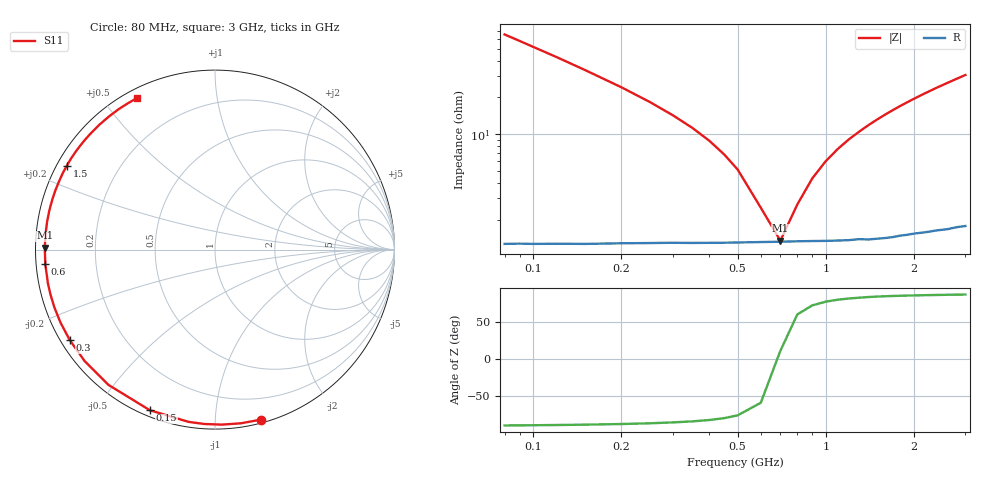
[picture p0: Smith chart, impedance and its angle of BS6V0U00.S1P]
! SIEMENS Small Signal Semiconductors
! BB640
! Si Tuning Diode in SOD323
! VR = 6 V
! S-Parameters:  July  1993
# GHz  S  MA  R  50
!  f  S11
! GHz  MAG  ANG
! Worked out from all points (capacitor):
!   33 points, 80 MHz to 3 GHz, reference 50 ohm
!   read as one part to ground: C = 30 pF near 80 MHz
!   lowest |Z| = 1.35 ohm at 700 MHz (marker M1)
!   series resonance near 689.1 MHz, so ESL is about 1.8 nH
!   S11 on the Smith chart (normalised r, x): 80 MHz: 0.03, -1.31; 150 MHz: 0.03, -0.67; 300 MHz: 0.03, -0.29; 600 MHz: 0.03, -0.04; 1.5 GHz: 0.03, +0.26; 3 GHz: 0.04, +0.61
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0.08  0.9815 -74.7
0.09  0.9785 -81.5
0.1  0.9759 -87.8
0.11  0.9734 -93.5
0.12  0.9711 -98.7
0.15  0.9657 -112.1
0.2  0.9593 -128.2
0.25  0.9556 -139.6
0.3  0.9532 -148.1
0.35  0.952 -154.7
0.4  0.951 -160.1
0.45  0.9503 -164.7
0.5  0.9497 -168.6
0.6  0.9489 -175.1
0.7  0.9485 179.4
0.8  0.9482 174.7
0.9  0.9482 170.5
1  0.9484 166.6
1.2  0.9486 159.6
1.4  0.9491 153.4
1.5  0.949 150.5
1.6  0.949 147.7
1.8  0.9482 142.4
2  0.9479 137.5
2.2  0.9482 132.9
2.4  0.9482 128.6
2.8  0.9488 120.8
3  0.9495 117.2
